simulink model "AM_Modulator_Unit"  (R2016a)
settings: Solver=ode3  StartTime=0.0  StopTime=1  FixedStep=1/5000000  RelTol=1e-3

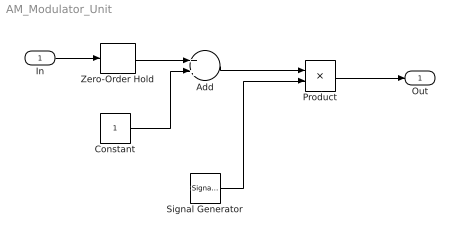
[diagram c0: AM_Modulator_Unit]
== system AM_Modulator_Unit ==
  In : Inport
  Add : Sum
  Constant : Constant
  Product : Product
  Signal Generator : SignalGenerator  Frequency=500000
  Zero-Order Hold : ZeroOrderHold  SampleTime=0.0000002
  Out : Outport
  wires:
  Constant/1 -> Add/2
  Add/1 -> Product/1
  In/1 -> Zero-Order Hold/1
  Zero-Order Hold/1 -> Add/1
  Signal Generator/1 -> Product/2
  Product/1 -> Out/1
